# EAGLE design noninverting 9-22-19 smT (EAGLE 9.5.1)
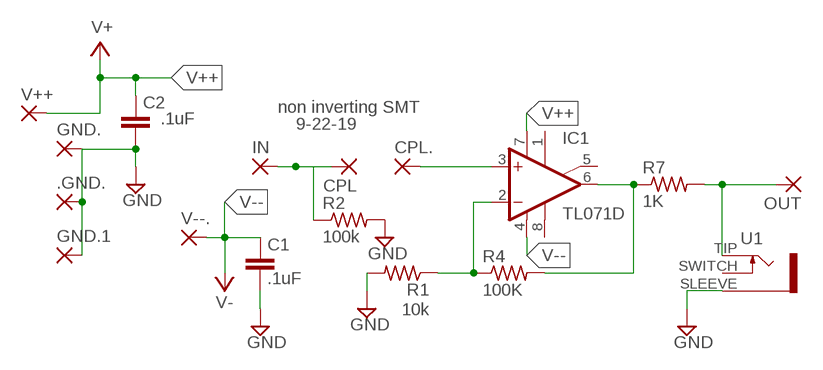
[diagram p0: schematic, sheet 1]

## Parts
.GND.  1,6/0,8  [1,6/0,8]
C1  .1uF  C-EU025-030X050  [C025-030X050]
C2  .1uF  C-EU025-030X050  [C025-030X050]
CPL  WIREPAD2,15/1,0  [2,15/1,0]
CPL.  WIREPAD2,15/1,0  [2,15/1,0]
GND.  WIREPAD2,15/1,0  [2,15/1,0]
GND.1  1,6/0,8  [1,6/0,8]
IC1  TL071D  [SO08]
IN  WIREPAD2,15/1,0  [2,15/1,0]
OUT  WIREPAD2,15/1,0  [2,15/1,0]
R1  10k  R-US_0207/2V  [0207/2V]
R2  100k  R-US_M1206  [M1206]
R4  100K  R-US_0207/2V  [0207/2V]
R7  1K  R-US_M1206  [M1206]
U1  35RAPC2AV  [35RAPCVAV]
V++2  V++  1,6/0,8  [1,6/0,8]
V--.  1,6/0,8  [1,6/0,8]

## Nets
GND: .GND..1(P) C1.2 C2.2 GND.1.1(P) GND..1(P) R1.2 R2.2 U1.SLEEVE
N$1: CPL.1(P) IN.1(P) R2.1
N$2: CPL..1(P) IC1.3(+IN)
N$5: IC1.6(OUT) R4.2 R7.1
N$19: OUT.1(P) R7.2 U1.TIP
N$20: IC1.2(-IN) R1.1 R4.1
V++: C2.1 IC1.7(V+) V++2.1(P) ; supply symbol labelled V+
V--: C1.1 IC1.4(V-) V--..1(P) ; supply symbol labelled V-
Unconnected: IC1.1(ON1) IC1.5(ON2) IC1.8(OPT) U1.SWITCH

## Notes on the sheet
- non inverting SMT
- 9-22-19

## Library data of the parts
.GND. GND.1 V++2 V--. = wirepad-NONAMES:1,6/0,8: THROUGH-HOLE PAD
C1 C2 = rcl:C-EU: CAPACITOR, European symbol; SPICEPREFIX: C
CPL CPL. GND. IN OUT = wirepad:WIREPAD: Wire PAD connect wire on PCB
IC1 = linear:TL071: OP AMP
R1 R2 R4 R7 = rcl:R-US_: RESISTOR, American symbol; SPICEPREFIX: R
U1 = MusicThingModular-CL:35RAPC2AV: Switchcraft 35RAPC2AV jack

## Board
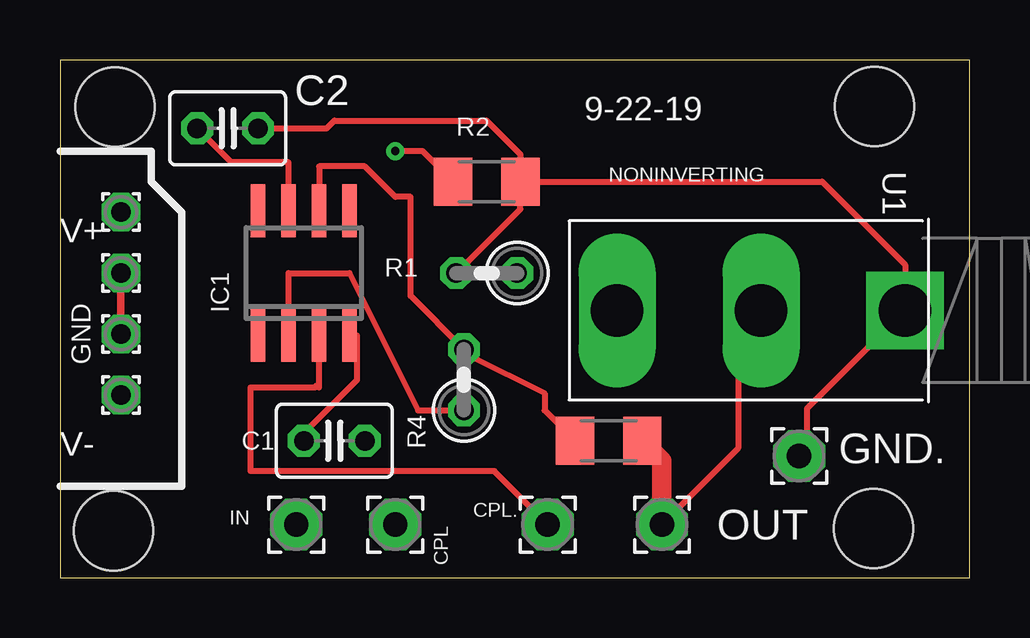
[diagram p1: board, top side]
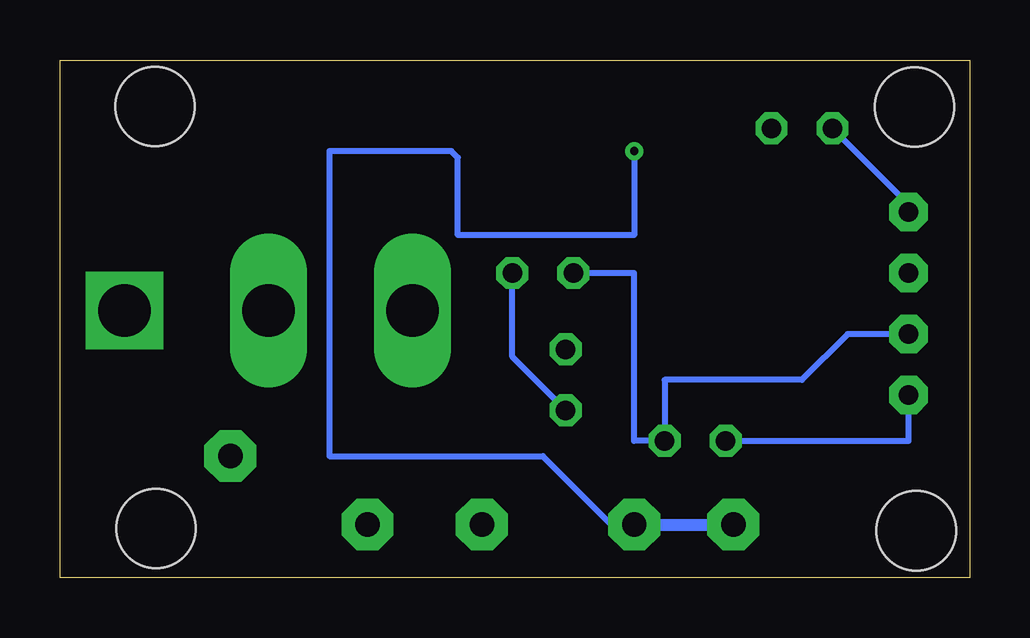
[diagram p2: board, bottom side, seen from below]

Size 37.9 x 21.58 mm. Coordinates in mm from the lower left corner, seen from the top.
Outline: 0,0 37.9,0 37.9,21.58 0,21.58 0,0
Copper layers (1*16): Top 0.035mm / dielectric 1.5mm / Bottom 0.035mm
Design rules "default": minimum track width 6mil, minimum drill 0.35mm, track to track 6mil, track to pad 6mil, pad to pad 6mil, via to via 6mil, smd to smd 6mil, copper to edge 40mil, drill to drill 6mil, minimum pad ring 10mil, minimum via ring 8mil, stop-mask expansion 4mil, vias tented up to drill 0mil, thermal gap 10mil
Holes 3.3 mm at 2.22,1.97 2.29,19.62 33.93,19.65 33.9,2.06

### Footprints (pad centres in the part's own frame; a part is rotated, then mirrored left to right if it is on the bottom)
1,6/0,8 = drill 0.813 pad 1.6 octagon: 1 0,0
C025-030X050 = drill 0.813 octagon: 1 -1.27,0; 2 1.27,0
2,15/1,0 = drill 1.016 pad 2.159 octagon: 1 0,0
SO08 = smd 0.6 x 2.2: 1 -1.905,-2.6; 2 -0.635,-2.6; 3 0.635,-2.6; 4 1.905,-2.6; 5 1.905,2.6; 6 0.635,2.6; 7 -0.635,2.6; 8 -1.905,2.6
0207/2V = drill 0.813 octagon: 1 -1.27,0; 2 1.27,0
M1206 = smd 1.6 x 2: 1 -1.4,0; 2 1.4,0
35RAPCVAV = drill 2.2 pad 1.778 square: SLEEVE 0,-6 | drill 2.2 pad 2.184 long: SWITCH 0,6; TIP 0,0

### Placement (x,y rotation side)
.GND.  2.54,12.7 0 top
C1  11.43,5.72 0 top
C2  6.98,18.73 0 top
CPL  13.97,2.22 270 top
CPL.  20.32,2.22 0 top
GND.  30.8,5.08 0 top
GND.1  2.54,10.16 0 top
IC1  10.16,12.7 0 top
IN  9.84,2.22 0 top
OUT  25.08,2.22 0 top
R1  17.78,12.7 180 top
R2  17.78,16.51 0 top
R4  16.83,8.26 90 top
R7  22.86,5.72 0 top
U1  29.21,11.15 90 top
V++2  2.54,15.24 0 top
V--.  2.54,7.62 0 top

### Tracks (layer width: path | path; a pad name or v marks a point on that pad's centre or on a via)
GND
  Top 0.254: C2.2 11.11,18.73 11.43,19.05 17.78,19.05 19.18,17.65 R2.2 | R2.2 31.75,16.51 35.21,13.05 U1.SLEEVE 31.11,7.05 31.11,5.4 GND..1 | R1.2 19.18,15.37 R2.2
  Top 0.305: GND.1.1 .GND..1
  Bottom 0.254: GND.1.1 5.08,10.16 6.98,8.26 12.7,8.26 C1.2 13.97,5.72 13.97,12.7 R1.2
N$1  (via drill 0.35)
  Top 0.254: R2.1 15.11,17.78 v13.97,17.78
  Bottom 0.254: CPL.1 14.45,1.75 17.78,5.08 26.67,5.08 26.67,17.78 21.59,17.78 21.32,17.51 21.32,14.29 13.97,14.29 v13.97,17.78
  Bottom 0.508: CPL.1 IN.1
N$2
  Top 0.254: IC1.3 10.79,7.94 10.71,8.03 10.62,7.94 7.94,7.94 7.94,4.45 18.1,4.45 CPL..1
N$5
  Top 0.254: R7.1 20.19,6.98 20.19,7.69 17.14,9.21 R4.2 14.6,11.75 14.6,15.88 13.97,15.88 12.7,17.15 10.79,17.15 IC1.6
N$19
  Top 0.254: OUT.1 28.26,5.4 28.26,10.19 U1.TIP
  Top 0.813: OUT.1 25.08,4.89 R7.2
N$20
  Top 0.254: IC1.2 9.53,12.7 12.06,12.7 14.92,6.98 R4.1
  Bottom 0.254: R4.1 19.05,9.21 R1.1
V++
  Top 0.254: IC1.7 9.53,17.31 7.13,17.31 | 7.13,17.31 | 7.13,17.31 C2.1
  Bottom 0.254: C2.1 2.54,15.56 V++2.1
V--
  Top 0.254: C1.1 10.16,6.03 12.38,8.26 12.38,10.1 IC1.4
  Bottom 0.254: C1.1 2.54,5.72 V--..1

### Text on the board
tNames: 9-22-19 | NONINVERTING | V+ | GND | V-
tValues: MICROGAIN!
